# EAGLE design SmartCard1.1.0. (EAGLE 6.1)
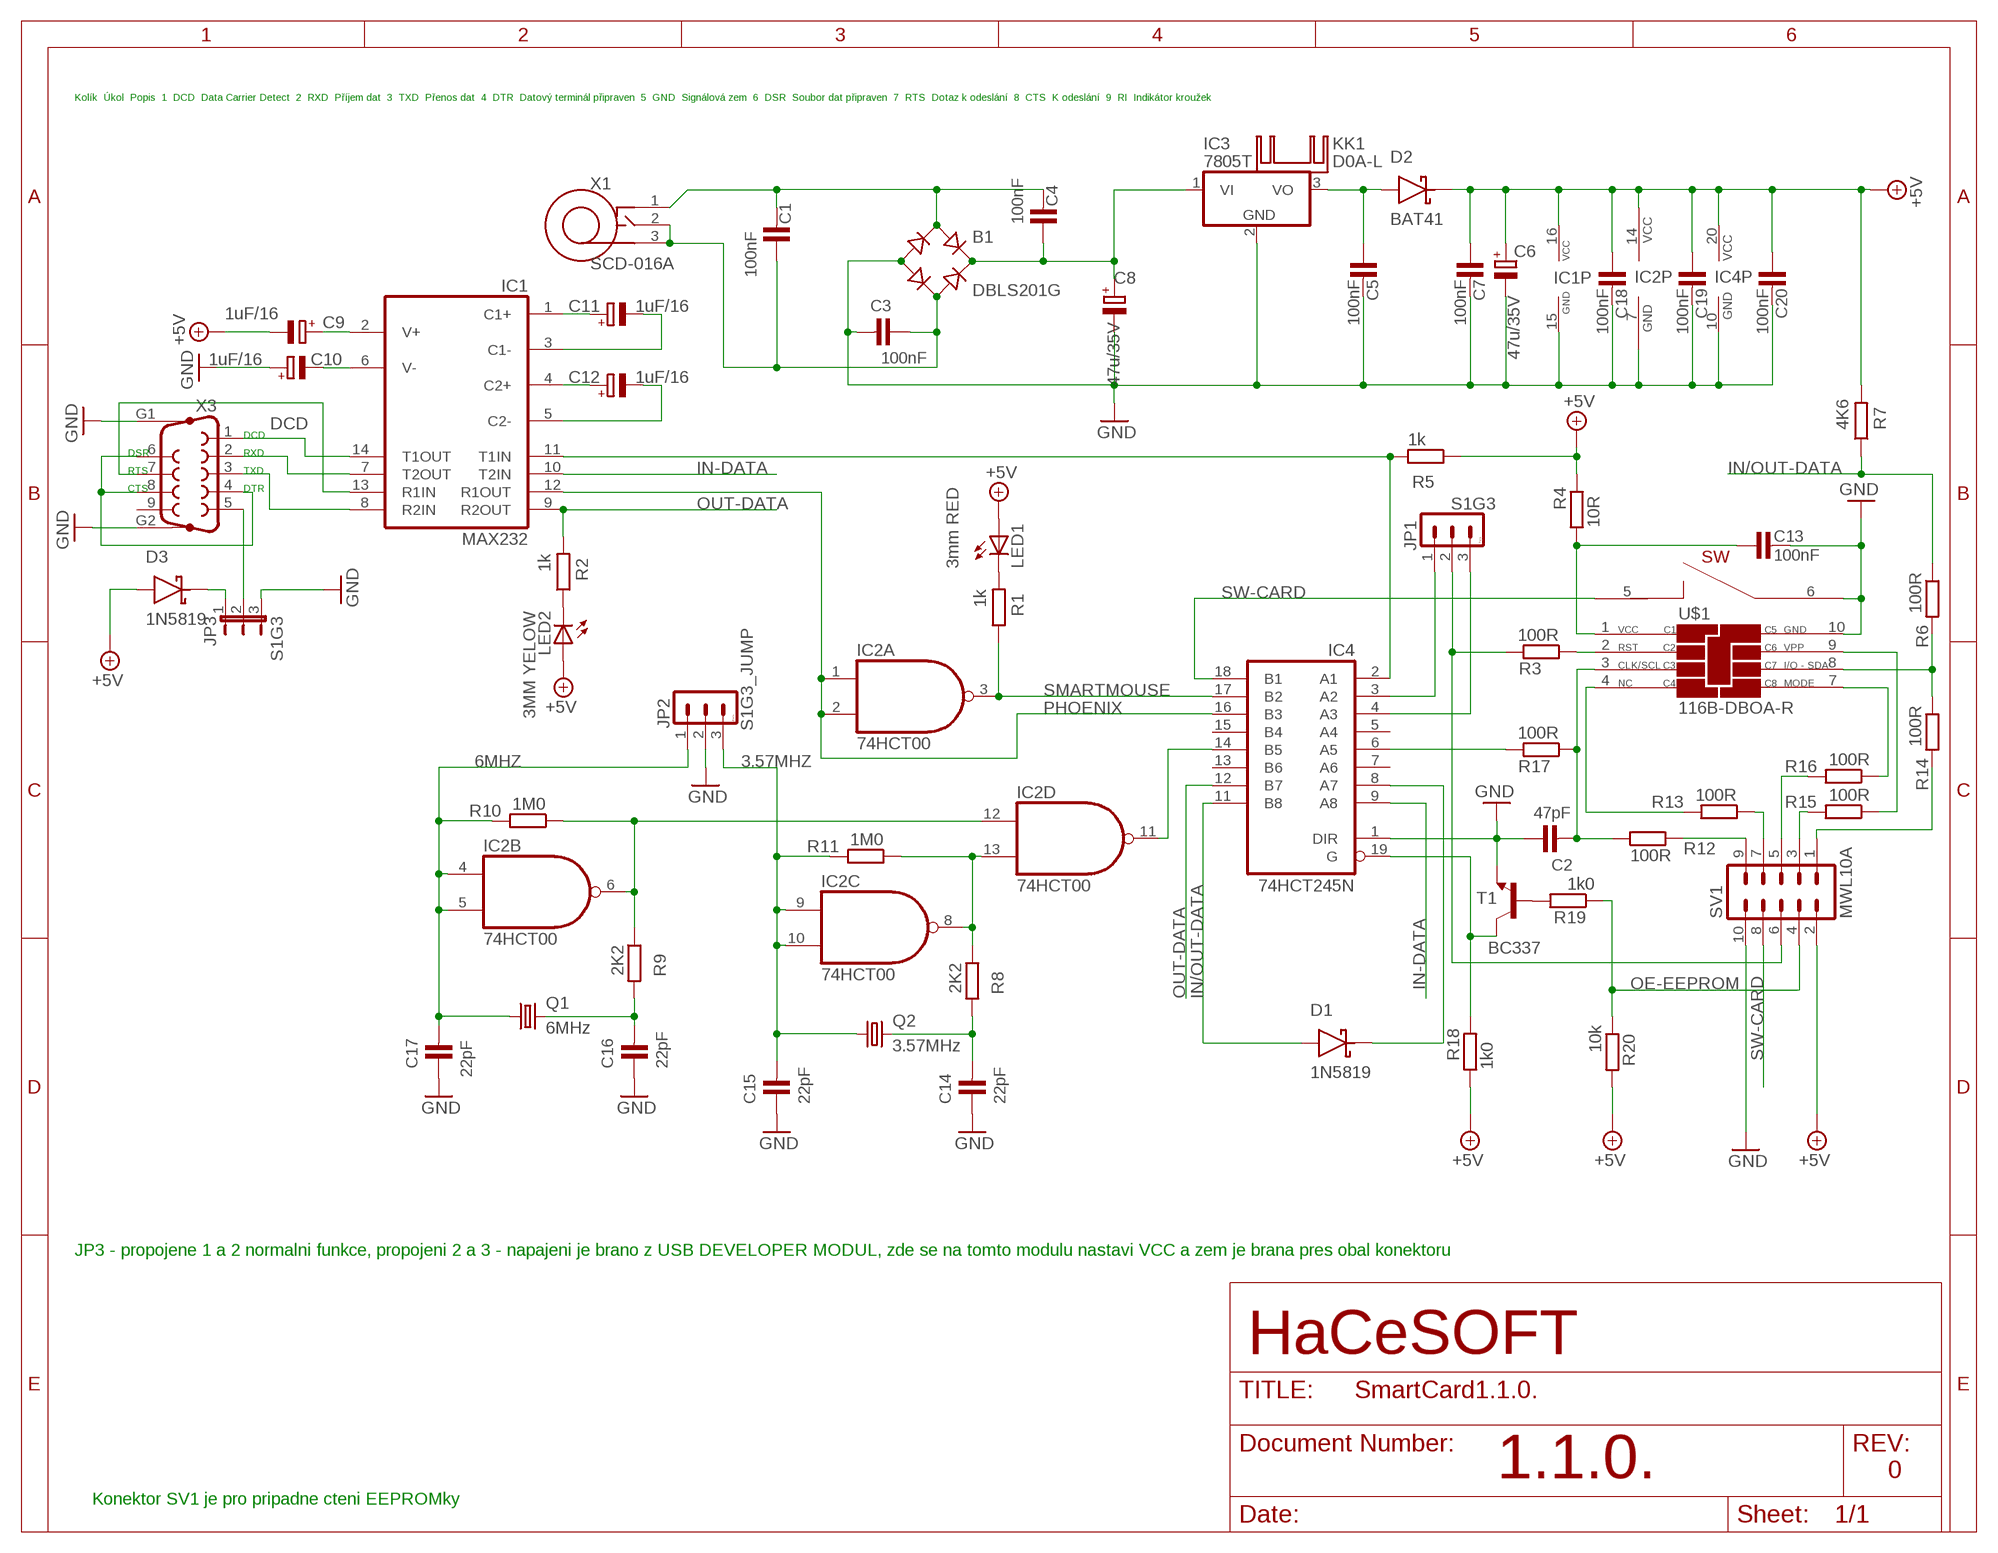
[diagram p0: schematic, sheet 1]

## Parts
B1  DBLS201G  [DBS]
C1  100nF  C-KERAMIK_SMD_1206  [1206]
C2  47pF  C-KERAMIK_SMD_1206  [1206]
C3  100nF  C-KERAMIK_SMD_1206  [1206]
C4  100nF  C-KERAMIK_SMD_1206  [1206]
C5  100nF  C-KERAMIK_SMD_1206  [1206]
C6  47u/35V  CPOL-EUE2.5-5  [E2,5-5]
C7  100nF  C-KERAMIK_SMD_1206  [1206]
C8  47u/35V  CPOL-EUE2.5-5  [E2,5-5]
C9  1uF/16  CPOL-EUSMCB  [SMC_B]
C10  1uF/16  CPOL-EUSMCB  [SMC_B]
C11  1uF/16  CPOL-EUSMCB  [SMC_B]
C12  1uF/16  CPOL-EUSMCB  [SMC_B]
C13  100nF  C-KERAMIK_SMD_1206  [1206]
C14  22pF  C-KERAMIK_SMD_1206  [1206]
C15  22pF  C-KERAMIK_SMD_1206  [1206]
C16  22pF  C-KERAMIK_SMD_1206  [1206]
C17  22pF  C-KERAMIK_SMD_1206  [1206]
C18  100nF  C-KERAMIK_SMD_1206  [1206]
C19  100nF  C-KERAMIK_SMD_1206  [1206]
C20  100nF  C-KERAMIK_5  [C-5]
D1  1N5819  BAT47  [DO35]
D2  BAT41  BAT47  [DO35]
D3  1N5819  BAT47  [DO35]
IC1  MAX232  [DIL16]
IC2  74HCT00  7400N  [DIL14]
IC3  7805T  [TO220H]
IC4  74HCT245N  [DIL20]
JP1  S1G3  S1G3_JUMP  [S1G3_JUM]
JP2  S1G3_JUMP  [S1G3_JUM]
JP3  S1G3  JP2E  [JP2]
KK1  D0A-L  [D02A-L]
LED1  3mm RED  LED3MM  [LED3MM]
LED2  3MM YELOW  LED3MM  [LED3MM]
Q1  6MHz  CSM-7X-DU  [CSM-7X-DU]
Q2  3.57MHz  CSM-7X-DU  [CSM-7X-DU]
R1  1k  R-EU_M1206  [M1206]
R2  1k  R-EU_0204/7  [0204/7]
R3  100R  R-EU_0204/7  [0204/7]
R4  10R  R-EU_0204/7  [0204/7]
R5  1k  R-EU_M1206  [M1206]
R6  100R  R-EU_M1206  [M1206]
R7  4K6  R-EU_0204/7  [0204/7]
R8  2K2  R-EU_M1206  [M1206]
R9  2K2  R-EU_M1206  [M1206]
R10  1M0  R-EU_M1206  [M1206]
R11  1M0  R-EU_M1206  [M1206]
R12  100R  R-EU_0204/7  [0204/7]
R13  100R  R-EU_0204/7  [0204/7]
R14  100R  R-EU_M1206  [M1206]
R15  100R  R-EU_M1206  [M1206]
R16  100R  R-EU_M1206  [M1206]
R17  100R  R-EU_0204/7  [0204/7]
R18  1k0  R-EU_M1206  [M1206]
R19  1k0  R-EU_0204/7  [0204/7]
R20  10k  R-EU_M1206  [M1206]
SV1  MWL10A  ML10L  [ML10L]
T1  BC337  [TO92]
U$1  116B-DBOA-R  [693030010810]
X1  SCD-016A  NAPAJECI_KONEKTOR_SCD-016A  [NAPAJECI_KONEKTOR_SCD-016A]
X3  F09HP  [F09HP]

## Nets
3.57MHZ: C15.2 IC2.9(C:I0) IC2.10(C:I1) JP2.3 Q2.1 R11.2
6MHZ: C17.2 IC2.4(B:I0) IC2.5(B:I1) JP2.1 Q1.1 R10.2
+5V: C6.+ C7.1 C9.- C18.1 C19.1 C20.1 D2.K D3.A IC1.16(VCC) IC2.14(P:VCC) IC4.20(VCC) LED1.A LED2.A R4.2 R5.1 R7.2 R18.1 R20.2 SV1.2
DCD: IC1.14(T1OUT) X3.1
DTR: X3.4 X3.6 X3.8
GND: B1.- C2.1 C3.2 C5.2 C6.- C7.2 C8.- C10.+ C13.2 C14.1 C15.1 C16.1 C17.1 C18.2 C19.2 C20.2 IC1.15(GND) IC2.7(P:GND) IC3.2(GND) IC4.1(DIR) IC4.10(GND) JP2.2 JP3.3 SV1.10 T1.1(E) U$1.6(SWITCH2) U$1.10(GND) X3.G1 X3.G2
IN-DATA: IC1.10(T2IN) IC4.9(A8)
IN/OUT-DATA: D1.A IC4.11(B8) R6.1 R7.1
IN/OUT-DATA-X: D1.K IC4.8(A7)
N$5: IC1.13(R1IN) X3.7
N$6: JP3.2 X3.5
N$7: B1.+ C4.1 C8.+ IC3.1(VI)
N$8: C9.+ IC1.2(V+)
N$9: B1.AC1 C1.2 C4.2 X1.1(OBAL)
N$10: D3.K JP3.1
N$11: C5.1 D2.A IC3.3(VO)
N$12: C10.- IC1.6(V-)
N$13: C11.+ IC1.1(C1+)
N$14: C12.+ IC1.4(C2+)
N$15: C11.- IC1.3(C1-)
N$16: C12.- IC1.5(C2-)
N$17: LED1.K(C) R1.2
N$19: IC4.19(G) R18.2 T1.3(C)
N$20: LED2.K(C) R2.1
N$21: JP1.2 R3.2 SV1.6
N$22: R3.1 U$1.2(RST)
N$23: IC4.3(A2) JP1.1
N$24: R6.2 R14.1 U$1.8(I/O-SDA)
N$25: IC1.11(T1IN) IC4.2(A1) R5.2
N$26: IC2.11(D:O) IC4.14(B5)
N$27: IC2.6(B:O) IC2.12(D:I0) R9.1 R10.1
N$28: C16.2 Q1.2 R9.2
N$29: C2.2 R12.1 R17.1 U$1.3(CLK/SCL)
N$30: IC2.8(C:O) IC2.13(D:I1) R8.1 R11.1
N$31: C14.2 Q2.2 R8.2
N$32: R12.2 SV1.9
N$33: R19.2 T1.2(B)
N$34: C13.1 R4.1 U$1.1(VCC)
N$35: R13.1 SV1.7
N$36: R13.2 U$1.4(NC)
N$37: R14.2 SV1.1
N$38: R15.1 U$1.9(VPP)
N$39: R16.1 U$1.7(MODE)
N$40: R15.2 SV1.3
N$41: R16.2 SV1.5
N$42: B1.AC2 C1.1 C3.1 X1.2 X1.3(PROSTREDEK)
N$43: IC4.4(A3) JP1.3
N$46: IC4.6(A5) R17.2
OE-EEPROM: R19.1 R20.1 SV1.4
OUT-DATA: IC1.9(R2OUT) IC4.12(B7) R2.2
PHOENIX: IC1.12(R1OUT) IC2.1(A:I0) IC2.2(A:I1) IC4.16(B3)
RXD: IC1.7(T2OUT) X3.2
SMARTMOUSE: IC2.3(A:O) IC4.17(B2) R1.1
SW-CARD: IC4.18(B1) SV1.8 U$1.5(SWITCH1)
TXD: IC1.8(R2IN) X3.3
Unconnected: IC4.5(A4) IC4.7(A6) IC4.13(B6) IC4.15(B4) X3.9

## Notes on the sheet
- Kolík  Úkol  Popis  1  DCD  Data Carrier Detect  2  RXD  Příjem dat  3  TXD  Přenos dat  4  DTR  Datový terminál připraven  5  GND  Signálová zem  6  DSR  Soubor dat připraven  7  RTS  Dotaz k odeslání  8  CTS  K odeslání  9  RI  Indikátor kroužek
- DCD
- DSR | RXD
- RTS | TXD
- CTS | DTR
- JP3 - propojene 1 a 2 normalni funkce, propojeni 2 a 3 - napajeni je brano z USB DEVELOPER MODUL, zde se na tomto modulu nastavi VCC a zem je brana pres obal konektoru
- HaCeSOFT
- 1.1.0. | 0
- Konektor SV1 je pro pripadne cteni EEPROMky

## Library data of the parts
B1 = rectifier:DB?*G: Single Phase 1.0 AMP Glass Passivated Bridge Rectifier Taiwan Semiconductor Co.,Ltd. - TSC Source: http://www.taiwansemi.com/TSCbig5/ezcatfiles/cust/img/img/db101g.pdf http://www.ts.com.tw/db/pictures/modules/PDT/PDT060207001/DBLS201G.pdf
C1-C5 C7 C13-C20 = #hacesoft:C-KERAMIK: Kondenzator - keramicky
C6 C8-C12 = rcl:CPOL-EU: POLARIZED CAPACITOR, European symbol
D1-D3 = #_GM99:BAT47
IC1 = maxim:MAX232: RS232 TRANSEIVER; MF: MAXIM; MPN: MAX232ACPE+; OC_FARNELL: 9723773; OC_NEWARK: 68K4544
IC2 = 74xx-us:74*00: Quad 2-input NAND gate
IC3 = linear:78*: Positive VOLTAGE REGULATOR Source: http://cache.national.com/ds/LM/LM78L05.pdf http://www.fairchildsemi.com/ds/LM/LM7805.pdf
IC4 = 74xx-eu:74*245: Octal BUS TRANSCEIVER, 3-state
JP1 JP2 = #PaJa_konektory:S1G3_JUMP: Radove konektory - koliky - 3x
JP3 = #hacesoft:JP2E: JUMPER
KK1 = heatsink:D0A-L: HEATSINK
LED1 LED2 = led:LED: LED
Q1 Q2 = crystal:CSM-7X-DU: SMD CRYSTAL; OC_FARNELL: unknown; OC_NEWARK: unknown
R1-R20 = resistor:R-EU_: RESISTOR, European symbol
SV1 = con-ml:ML10L: HARTING; OC_FARNELL: unknown; OC_NEWARK: unknown
T1 = transistor:BC337: NPN TRANSISTOR
U$1 = Smart Card Socket Through Hole Type, Single Port:116B-DBOA-R
X1 = #hacesoft:NAPAJECI_KONEKTOR_SCD-016A
X3 = con-subd:F09HP: SUB-D; OC_FARNELL: unknown; OC_NEWARK: unknown

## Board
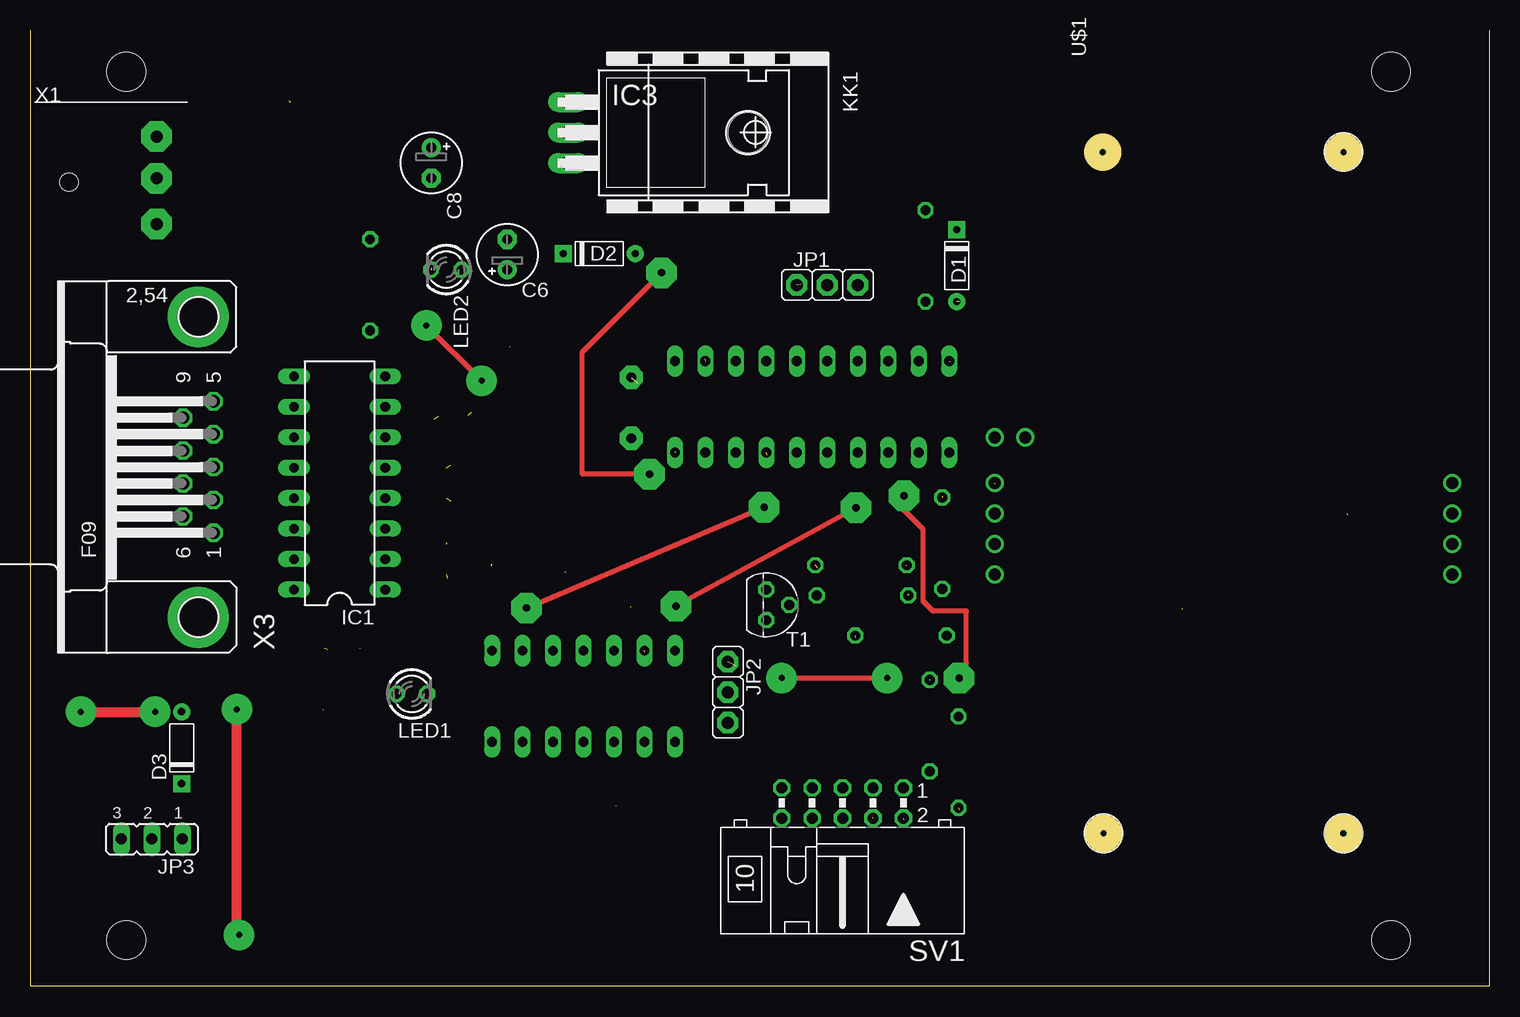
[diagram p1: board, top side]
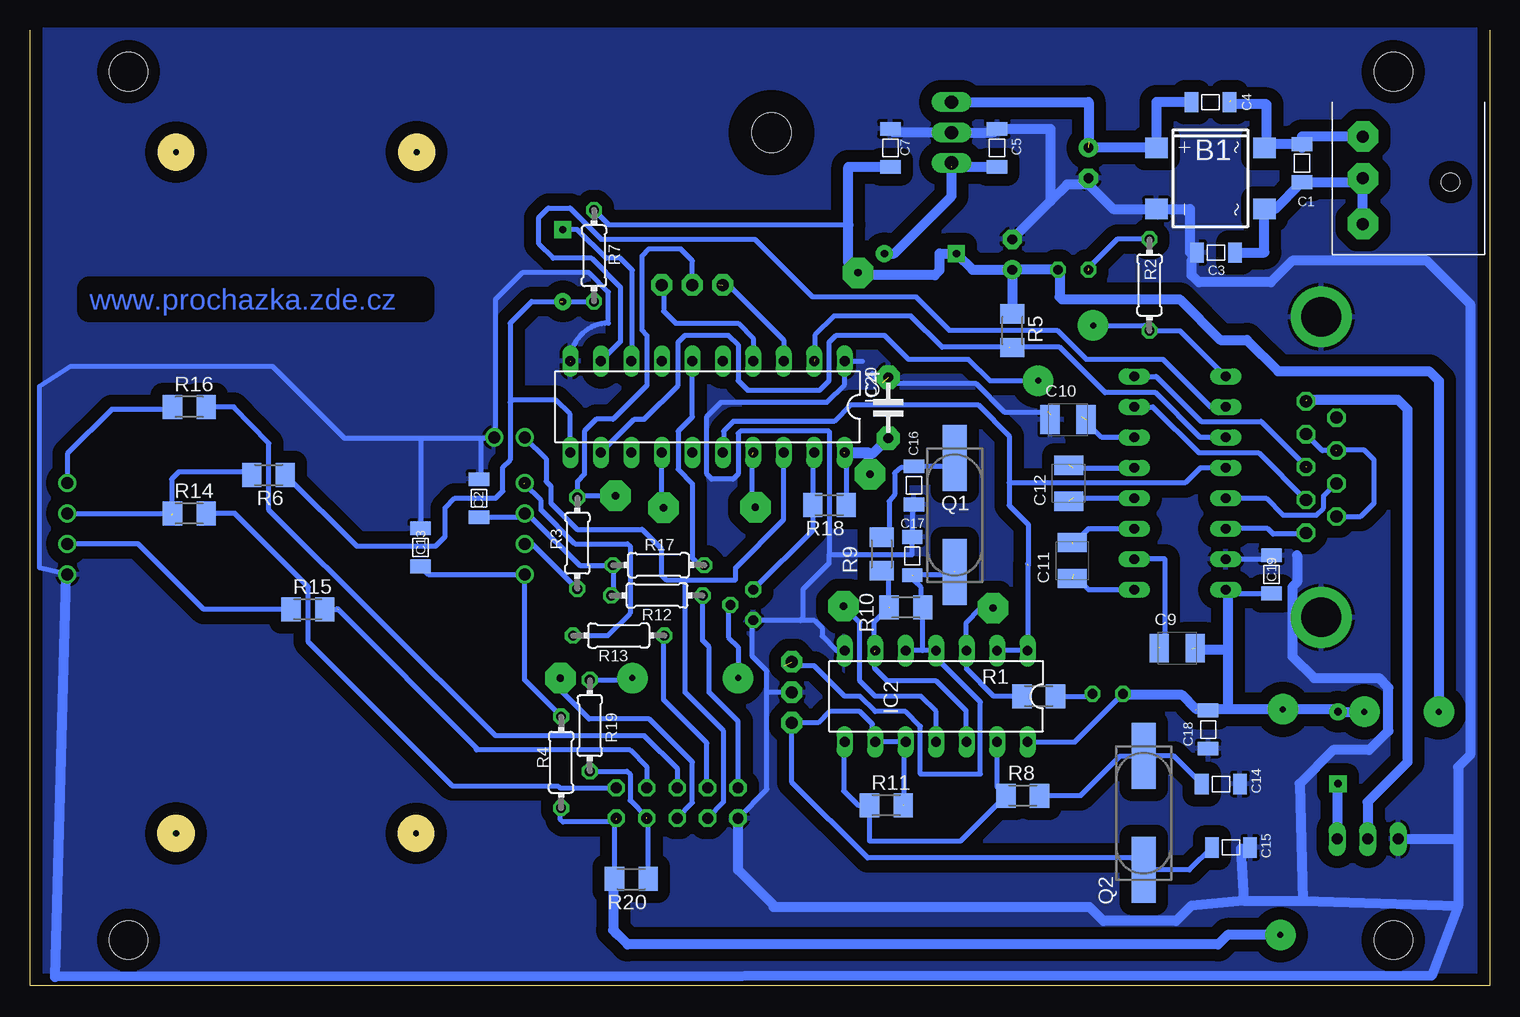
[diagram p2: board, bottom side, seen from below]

Size 121.63 x 79.68 mm. Coordinates in mm from the lower left corner, seen from the top.
Outline: 121.63,79.68 121.63,0 0,0 0,79.68
Copper layers (1*16): Top 0.035mm / dielectric 1.5mm / Bottom 0.035mm
Design rules: minimum track width 10mil, minimum drill 12mil, track to track 8mil, track to pad 8mil, pad to pad 8mil, via to via 8mil, smd to smd 8mil, copper to edge 40mil, drill to drill 8mil, minimum pad ring 10mil, minimum via ring 8mil, stop-mask expansion 4mil, vias tented up to drill 0mil, thermal gap 10mil
Holes 3.2 mm at 113.43,3.81 113.43,76.2 8.02,3.81 8.02,76.2

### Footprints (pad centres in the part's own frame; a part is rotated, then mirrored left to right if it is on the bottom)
DBS = smd 1.7 x 1.9: + -2.55,-4.5; - 2.55,-4.5; AC1 -2.55,4.5; AC2 2.55,4.5
1206 = smd 1.143 x 1.702: 1 -1.587,0; 2 1.587,0
E2,5-5 = drill 0.813 pad 1.6: + -1.27,0 | drill 0.813 pad 1.6 octagon: - 1.27,0
SMC_B = smd 1.6 x 2.4: + -1.5,0; - 1.5,0
C-5 = drill 0.813 pad 1.93 octagon: 1 -2.54,0; 2 2.54,0
DO35 = drill 0.61 pad 1.422: A 6,0 | drill 0.61 pad 1.422 square: K 0,0
DIL16 = drill 0.813 long: 1 -8.89,-3.81; 2 -6.35,-3.81; 3 -3.81,-3.81; 4 -1.27,-3.81; 5 1.27,-3.81; 6 3.81,-3.81; 7 6.35,-3.81; 8 8.89,-3.81; 9 8.89,3.81; 10 6.35,3.81; 11 3.81,3.81; 12 1.27,3.81; 13 -1.27,3.81; 14 -3.81,3.81; 15 -6.35,3.81; 16 -8.89,3.81
DIL14 = drill 0.813 long: 1 -7.62,-3.81; 2 -5.08,-3.81; 3 -2.54,-3.81; 4 0,-3.81; 5 2.54,-3.81; 6 5.08,-3.81; 7 7.62,-3.81; 8 7.62,3.81; 9 5.08,3.81; 10 2.54,3.81; 11 0,3.81; 12 -2.54,3.81; 13 -5.08,3.81; 14 -7.62,3.81
TO220H = drill 1.118 long: 1 -2.54,-10.16; 2 0,-10.16; 3 2.54,-10.16 | hole 3.302: 0,4.826
DIL20 = drill 0.813 long: 1 -11.43,-3.81; 2 -8.89,-3.81; 3 -6.35,-3.81; 4 -3.81,-3.81; 5 -1.27,-3.81; 6 1.27,-3.81; 7 3.81,-3.81; 8 6.35,-3.81; 9 8.89,-3.81; 10 11.43,-3.81; 11 11.43,3.81; 12 8.89,3.81; 13 6.35,3.81; 14 3.81,3.81; 15 1.27,3.81; 16 -1.27,3.81; 17 -3.81,3.81; 18 -6.35,3.81; 19 -8.89,3.81; 20 -11.43,3.81
S1G3_JUM = drill 1.016 pad 1.778 octagon: 1 -2.54,0; 2 0,0; 3 2.54,0
JP2 = drill 0.914 long: 1 -2.54,0; 2 0,0; 3 2.54,0
LED3MM = drill 0.813 octagon: A -1.27,0; K 1.27,0
CSM-7X-DU = smd 5.5 x 2: 1 -4.75,0; 2 4.75,0
M1206 = smd 1.6 x 2: 1 -1.4,0; 2 1.4,0
0204/7 = drill 0.813 octagon: 1 -3.81,0; 2 3.81,0
ML10L = drill 0.914 octagon: 1 -5.08,-1.27; 2 -5.08,1.27; 3 -2.54,-1.27; 4 -2.54,1.27; 5 0,-1.27; 6 0,1.27; 7 2.54,-1.27; 8 2.54,1.27; 9 5.08,-1.27; 10 5.08,1.27
TO92 = drill 0.813 octagon: 1 1.27,0; 2 0,1.905; 3 -1.27,0
693030010810 = drill 1: 1 0,38.1; 2 2.54,38.1; 3 5.08,38.1; 4 7.62,38.1; 5 11.43,38.1; 6 11.43,35.56; 7 7.62,0; 8 5.08,0; 9 2.54,0; 10 0,0 | drill 0.5 pad 3: P$1 -21.594,29.048; P$2 -21.589,9.053; P$3 35.213,9.05; P$4 35.213,29.097
NAPAJECI_KONEKTOR_SCD-016A = drill 1 pad 2.54 octagon: 1 0,7.303; 2 0,3.81; 3 0,0 | hole 1.5: -7.303,3.493
F09HP = drill 1.016 octagon: 1 -5.486,-1.27; 2 -2.743,-1.27; 3 0,-1.27; 4 2.743,-1.27; 5 5.486,-1.27; 6 -4.115,1.27; 7 -1.372,1.27; 8 1.372,1.27; 9 4.115,1.27 | drill 3.302 pad 5.08: G1 -12.522,0; G2 12.522,0

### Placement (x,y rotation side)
B1  23.26,67.31 270 bottom
C1  15.64,68.58 90 bottom
C2  84.22,40.64 270 bottom
C3  22.8,61.12 180 bottom
C4  23.26,73.66 0 bottom
C5  41.04,69.85 90 bottom
C6  39.77,60.96 90 top
C7  49.93,69.85 90 bottom
C8  33.43,68.59 270 top
C9  26.03,28.14 0 bottom
C10  35.13,47.19 0 bottom
C11  34.78,35.44 90 bottom
C12  35.08,41.89 90 bottom
C13  89.09,36.54 90 bottom
C14  22.39,16.81 180 bottom
C15  21.54,11.53 180 bottom
C16  47.97,41.71 90 bottom
C17  48.11,35.82 270 bottom
C18  23.45,21.36 270 bottom
C19  18.18,34.29 90 bottom
C20  50.11,48.18 90 bottom
D1  77.23,63.04 270 top
D2  44.43,61.04 0 top
D3  12.63,16.84 90 top
IC1  25.8,41.91 90 top
IC2  46.12,24.13 180 bottom
IC3  55.01,71.12 270 top
IC4  65.17,48.26 180 bottom
JP1  66.44,58.42 0 top
JP2  58.15,24.46 270 top
JP3  10.16,12.23 180 top
KK1  55.01,71.12 180 top
LED1  31.82,24.33 0 top
LED2  34.69,59.69 180 top
Q1  44.58,39.24 90 bottom
Q2  28.83,14.39 90 bottom
R1  37.57,24.13 0 bottom
R2  28.34,58.42 270 bottom
R3  76.02,36.89 90 bottom
R4  77.37,18.63 270 bottom
R5  39.77,54.61 270 bottom
R6  101.75,42.58 180 bottom
R7  74.63,60.85 90 bottom
R8  38.9,15.84 0 bottom
R9  50.66,35.99 90 bottom
R10  48.64,31.53 0 bottom
R11  50.27,15.04 0 bottom
R12  69.38,32.53 0 bottom
R13  72.58,29.19 180 bottom
R14  108.35,39.37 0 bottom
R15  98.48,31.38 0 bottom
R16  108.35,48.26 0 bottom
R17  69.25,35.06 0 bottom
R18  55.01,40.06 180 bottom
R19  74.98,21.68 90 bottom
R20  71.52,8.89 180 bottom
SV1  67.71,15.24 180 top
T1  61.36,31.75 270 top
U$1  118.51,34.29 90 top
X1  10.56,63.5 0 top
X3  14.03,43.24 90 top

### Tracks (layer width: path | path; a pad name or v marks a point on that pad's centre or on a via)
3.57MHZ  (1 unrouted)
  Bottom 0.406: 48.83,15.04 48.83,20.15 IC2.10 IC2.9 51.43,20.55 51.43,21.82 52.47,22.86 55.01,22.86 55.95,21.92 JP2.3 58.15,16.96 51.83,10.64 29.83,10.64 Q2.1 25.02,9.64 C15.2
6MHZ  (3 unrouted)
  Bottom 0.406: IC2.4 IC2.5 48.83,27.94 48.83,27.84 | JP2.1 57.99,26.84 | IC2.4 46.12,27.33 42.43,23.64 42.43,17.64 47.43,17.64 47.43,21.63 48.66,22.86 51.2,22.86 52.47,24.13 53.74,24.13 56.28,26.67 58.82,26.67 | IC2.4 47.24,27.94 R10.2 47.38,31.67 47.38,33.19 47.98,33.79 47.98,34.14 48.03,34.19 47.93,34.29 44.68,34.29 44.63,34.34 44.63,34.49
+5V  (via drill 0.5 pad 2.54, 0.6 pad 2.54)  (5 unrouted)
  Top 0.406: v51.63,42.64 46.03,42.64 46.03,52.84 v52.63,59.44
  Top 0.813: v4.23,22.84 v10.43,22.84 | v17.43,4.24 17.23,4.24 v17.23,23.04
  Bottom 0.406: IC1.16 21.99,32.7 C19.1 | R20.2 72.92,13.75 | 72.92,13.75 72.83,13.84 | 72.92,13.75 73.03,13.64 77.23,13.64 77.43,13.84 77.43,14.64 | C6.+ 39.83,59.63 | R5.1 40,56.24 | IC4.20 53.61,44.45 R18.1 | R7.2 73.41,63.44 53.43,63.44 | v51.63,42.64 51.43,42.84 | C18.1 24.48,22.95 24.48,23.14 | IC2.14 34.56,20.32 LED1.A 30.63,24.25 30.63,24.24
  Bottom 0.813: C7.1 53.41,68.26 53.43,68.24 53.43,63.44 53.43,60.24 v52.63,59.44 53.43,59.24 46.23,59.24 45.83,59.64 45.83,61.04 D2.K 43.08,59.69 C6.+ 36.06,59.69 36.01,59.64 | LED2.A 36.01,59.64 | 39.83,59.63 39.77,59.57 R5.1 | 36.01,59.64 35.83,59.46 35.83,57.44 35.63,57.24 25.83,57.24 22.43,53.84 20.23,53.84 17.63,51.24 5.03,51.24 4.23,50.44 v4.23,22.84 | v10.43,22.84 D3.A 12.83,23.04 v17.23,23.04 21.83,23.04 | 21.83,23.04 24.43,23.04 25.63,24.24 30.63,24.24 | 21.99,32.7 21.83,32.54 21.83,28.04 | 21.83,28.04 21.83,23.04 | 24.93,28.14 24.83,28.04 21.83,28.04 | R20.2 73.03,8.78 73.03,4.64 72.73,4.34 72.63,4.24 71.83,3.44 22.63,3.44 21.83,4.24 v17.43,4.24 | v51.63,42.64 51.73,42.64 51.73,44.44 53.83,44.44 53.83,44.39 51.36,44.39 C20.1
DCD
  Bottom 0.406: X3.1 15.41,37.64 18.03,37.64 18.49,38.1 IC1.14
DTR  (1 unrouted)
  Bottom 0.406: X3.6 10.75,39.12 9.63,40.24 9.63,43.84 10.43,44.64 12.83,44.64 | X3.8 13.93,44.61 X3.4
GND  (3 unrouted)
  Bottom 0.406: U$1.10 120.83,34.84 120.83,49.99 118.23,51.64 101.43,51.64 95.43,45.64 89.03,45.64 | 89.03,45.64 84.03,45.64 | 84.03,45.64 83.03,45.64 | 83.03,45.64 82.83,45.64 82.83,57.24 80.63,59.44 75.03,59.44 73.43,57.84 73.43,55.24 arc-90 76.63,52.04 | C13.2 89.03,38.19 89.03,45.64 | C2.1 84.03,42.42 84.03,45.64 | U$1.6 83.03,45.64 | 52.26,52.07 IC4.1 53.74,50.13 55.23,48.64 64.03,48.64 65.23,47.44 65.23,42.64 64.83,42.24 63.03,42.24 62.63,42.64 62.63,46.04 62.43,46.24 55.03,46.24 55.03,35.94 | 36.52,47.58 36.52,48.13 | 51.43,51.04 50.63,50.24 42.83,50.24 40.43,47.84 36.83,47.84 | SV1.10 60.23,16.37 60.23,24.44 | JP2.2 60.21,24.46 60.23,24.44 | 60.23,24.44 60.23,26.24 61.43,27.44 61.43,30.44 | 61.43,30.44 61.43,30.48 | 57.43,30.44 57.23,30.64 57.23,33.04 55.03,35.24 55.03,35.94 | 57.43,30.44 61.43,30.44 | 57.43,30.44 56.24,30.44 55.63,29.83 55.63,29.14 54.43,27.94 53.83,27.94 53.83,27.84 IC2.7 | IC1.15 18.18,35.56 C19.2 | 55.03,35.94 48.11,35.94 C17.1 48.11,40.12 C16.1 | C3.2 24.98,61.12 24.98,60.24 | 24.98,60.19 24.98,60.24 | 24.98,60.24 24.88,60.24 24.88,60.34
  Bottom 0.813: 20.72,11.43 20.47,7.09 | 20.47,7.09 15.58,7.09 | 15.58,7.09 2.63,6.64 | 24.83,60.44 24.83,59.24 24.23,58.64 18.23,58.64 16.43,60.44 5.23,60.44 1.63,56.84 1.63,19.24 2.63,18.24 2.63,12.04 | 59.63,6.64 62.63,9.64 62.63,13.84 | 2.63,6.64 4.83,0.84 119.53,0.74 118.63,34.24 | JP3.3 2.83,12.24 2.63,12.04 | 15.58,7.09 15.83,16.84 13.03,19.64 10.03,19.64 8.43,21.24 8.43,24.84 9.23,25.64 14.63,25.64 16.43,27.44 16.43,33.24 16.03,33.64 16.03,35.88 | 2.63,12.04 2.63,6.64 | 36.59,65.41 35.2,66.8 33.42,66.8 31.38,64.76 B1.- | 36.59,65.41 C6.- | C7.2 49.61,71.12 IC3.2 41.36,71.12 C5.2 36.59,71.44 36.59,65.41 | B1.- 27.43,64.76 27.43,64.69 | B1.- 24.98,64.76 24.98,61.12 | 20.47,7.09 24.88,6.64 26.13,5.39 32.18,5.39 33.33,6.54 59.68,6.54
  pour Bottom (isolate 1.016): 0.23,79.64 121.63,79.64 121.63,-0.16 0.23,-0.16
IN-DATA
  Bottom 0.406: IC4.9 72.43,53.7 72.43,58.24 74.83,60.64 78.03,60.64 79.23,61.84 79.23,64.04 78.43,64.84 76.63,64.84 74.03,62.24 61.23,62.24 56.43,57.44 47.83,57.44 45.03,54.64 36.03,54.64 33.63,52.24 27.23,52.24 23.25,48.26 IC1.10
IN/OUT-DATA  (1 unrouted)
  Bottom 0.406: R6.1 94.41,36.64 87.83,36.64 87.03,37.44 87.03,39.84 86.23,40.64 82.83,40.64 82.23,41.24 82.23,43.24 81.63,43.84 81.63,48.64 | 81.63,48.64 81.63,55.24 79.83,57.04 77.43,57.04 | IC4.11 76.63,44.48 76.63,47.64 77.83,48.84 81.43,48.84 81.63,48.64 | D1.A R7.1
IN/OUT-DATA-X
  Bottom 0.406: IC4.8 71.63,52.38 71.43,52.58 71.43,59.64 72.43,60.64 73.63,60.64 76.03,63.04 D1.K
N$5
  Bottom 0.406: IC1.13 18.63,40.64 17.23,39.24 14.43,39.24 13.83,39.84 13.83,40.84 12.8,41.87 X3.7
N$6  (1 unrouted)
  Bottom 0.813: JP3.2 10.16,15.31 6.83,18.64 6.83,48.04 7.63,48.84 15.23,48.84
N$7  (1 unrouted)
  Bottom 0.813: C4.1 27.76,73.66 B1.+ 32.92,69.86 33.42,70.36 33.42,73.66 IC3.1
N$8  (1 unrouted)
  Bottom 0.406: 27.47,28.14 27.03,28.58 27.03,35.56 IC1.2
N$9  (1 unrouted)
  Bottom 0.813: X1.1 15.64,70.8 C1.2 | C1.2 15.64,69.85 | C1.2 18.76,70.17 B1.AC1 18.58,69.86 18.58,73.49 21.58,73.49 21.58,73.79
N$10
  Bottom 0.813: D3.K 12.7,16.77 JP3.1
N$11  (1 unrouted)
  Bottom 0.813: C5.1 44.85,68.26 IC3.3 45.32,68.58 | D2.A 49.63,61.04 44.83,65.84 44.83,68.24 45.03,68.44 | 45.03,68.44 44.83,68.64 44.83,68.44 45.03,68.44
N$12  (1 unrouted)
  Bottom 0.406: IC1.6 32.31,45.72 34.03,47.44
N$13  (1 unrouted)
  Bottom 0.406: 34.69,34.29 33.42,33.02 IC1.1
N$14  (1 unrouted)
  Bottom 0.406: 34.69,40.64 IC1.4
N$15  (1 unrouted)
  Bottom 0.406: 34.69,36.83 33.42,38.1 IC1.3
N$16  (1 unrouted)
  Bottom 0.406: 34.69,43.18 IC1.5
N$17
  Bottom 0.406: R1.2 33.09,24.13 LED1.K
N$19
  Bottom 0.406: IC4.19 56.41,44.45 R18.2 56.41,37.97 T1.3
N$20  (2 unrouted)
  Bottom 0.406: 33.25,59.82 33.43,59.64 | R2.1 31.04,62.23 33.43,59.84
N$21  (via drill 0.6 pad 2.54)  (1 unrouted)
  Top 0.406: v77.43,25.64 78.03,26.84 78.03,31.24 75.23,31.24 74.43,32.04 74.43,38.04 72.83,39.64 v72.83,40.84
  Bottom 0.406: 66.63,58.61 JP1.2 66.43,60.44 67.43,61.44 70.03,61.44 70.63,60.84 70.63,54.64 70.23,54.24 70.23,50.04 73.03,47.24 74.43,47.24 75.43,46.24 75.43,42.64 76.02,42.05 R3.2 | SV1.6 66.43,15.25 66.43,18.64 70.03,22.24 75.03,22.24 77.23,24.44 v77.43,25.64 | v72.83,40.84 76.03,40.84
N$22
  Bottom 0.406: U$1.2 79.77,36.83 R3.1
N$23  (1 unrouted)
  Bottom 0.406: IC4.3 58.82,53.83 63.43,58.44 64.23,58.44
N$24  (1 unrouted)
  Bottom 0.406: U$1.8 R14.1 | R6.2 103.41,42.84 109.23,42.84 109.83,42.24 109.83,39.24
N$25  (2 unrouted)
  Bottom 0.406: IC1.11 24.11,45.72 27.83,49.44 32.03,49.44 35.83,53.24 40.03,53.24 | R5.2 39.77,53.04 39.97,53.24 45.63,53.24 48.23,55.84 54.63,55.84 56.23,54.24 56.23,52.24
N$26  (via drill 0.6 pad 2.54)
  Top 0.406: v53.83,31.64 v68.83,39.84
  Bottom 0.406: IC2.11 46.12,22.86 47.39,24.13 51.2,24.13 52.47,25.4 52.47,30.28 v53.83,31.64 | v68.83,39.84 68.98,39.99 IC4.14
N$27  (2 unrouted)
  Bottom 0.406: IC2.12 43.63,20.37 43.63,22.91 46.12,25.4 50.19,25.4 51.23,26.44 51.23,27.84 | IC2.6 51.28,27.94 51.28,30.34 50.13,31.49 50.13,31.54 50.08,31.59 50.08,34.44 50.51,34.44 R9.1
N$28
  Bottom 0.406: Q1.2 45.27,43.3 C16.2 47.58,43.19 49.03,43.19 49.58,42.74 49.58,40.94 50.03,40.39 50.03,37.44 50.13,37.34 50.61,37.34 R9.2
N$29  (2 unrouted)
  Bottom 0.406: U$1.3 80.41,39.05 | 80.41,39.05 C2.2 | 80.41,39.05 79.84,39.05 75.83,35.04 73.03,35.04 73.03,32.84 73.23,32.64
N$30
  Bottom 0.406: IC2.8 53.83,20.23 53.83,16.24 52.63,15.04 R11.1 51.67,12.08 51.63,12.04 44.1,12.04 R8.1 41.04,16.58 IC2.13
N$31
  Bottom 0.406: R8.2 34.09,15.84 30.79,19.14 Q2.2 26.31,19.14 C14.2
N$32
  Bottom 0.406: SV1.9 62.63,22.04 65.03,24.44 65.03,28.24 65.57,28.78 R12.2
N$33  (via drill 0.5 pad 2.54)  (1 unrouted)
  Top 0.406: v62.63,25.64 v71.43,25.64
  Bottom 0.406: T1.2 63.43,31.58 63.43,29.04 62.63,28.24 v62.63,25.64 | v71.43,25.64 71.63,25.44 75.03,25.44
N$34
  Bottom 0.406: C13.1 88.43,34.29 U$1.1 80.41,25.48 R4.1
N$35  (1 unrouted)
  Bottom 0.406: SV1.7 65.23,16.57 65.23,20.24 68.83,23.84 68.83,29.04
N$36  (1 unrouted)
  Bottom 0.406: 80.43,41.84 79.03,40.44 79.03,39.64 76.23,36.84 71.83,36.84 71.63,36.64 71.63,31.04 73.48,29.19 R13.2
N$37
  Bottom 0.406: 72.92,16.64 SV1.1 77.5,16.51 77.63,16.64 86.43,16.64 98.43,28.64 98.43,33.24 104.56,39.37 R14.2
N$38
  Bottom 0.406: R15.1 107.17,31.38 112.62,36.83 U$1.9
N$39
  Bottom 0.406: R16.1 109.97,48.04 114.83,48.04 118.51,44.36 U$1.7
N$40  (1 unrouted)
  Bottom 0.406: R15.2 95.97,31.38 | 96.03,31.44 84.43,19.84 84.43,19.64 71.63,19.64 70.25,18.26 SV1.3
N$41
  Bottom 0.406: R16.2 104.65,48.26 101.73,45.24 101.73,39.64 82.83,20.84 70.43,20.84 67.71,18.12 SV1.5
N$42
  Bottom 0.813: X1.3 X1.2 10.88,66.99 C1.1 17.87,64.76 B1.AC2 18.76,61.12 C3.1
N$43
  Bottom 0.406: JP1.3 68.83,58.27 68.83,56.24 67.83,55.24 62.63,55.24 61.36,53.97 IC4.4
N$46  (1 unrouted)
  Bottom 0.406: IC4.6 66.44,47.43 67.63,46.24 67.63,43.04 66.43,41.84 66.43,35.64 65.63,34.84 | 65.44,35.45 R17.2
OE-EEPROM  (1 unrouted)
  Bottom 0.406: R20.1 70.12,13.84 SV1.4 | R19.1 71.86,17.87 71.63,17.64 71.63,15.44 70.23,14.04 70.23,13.84
OUT-DATA  (via drill 0.5 pad 2.54)
  Top 0.406: v37.63,50.44 v33.03,55.04
  Bottom 0.406: 22.12,50.8 IC1.9 25.8,54.61 R2.2 28.77,55.04 v33.03,55.04 | IC4.12 71.27,47.24 70.43,47.24 67.63,50.04 67.63,53.64 67.03,54.24 63.43,54.24 62.63,53.44 62.63,50.44 61.83,49.64 55.83,49.64 55.03,50.44 55.03,53.64 54.43,54.24 50.43,54.24 48.43,52.24 43.43,52.24 41.63,50.44 v37.63,50.44
PHOENIX  (1 unrouted)
  Bottom 0.406: IC2.2 IC2.1 38.5,35.17 | IC1.12 24.09,43.18 25.36,41.91 40.03,41.91 | 40.03,41.91 40.03,45.84 42.63,48.44 53.23,48.44 54.63,47.04 63.03,47.04 63.83,46.24 63.83,44.52 IC4.16 | 40.03,41.91 40.03,40.04 38.43,38.44 38.43,35.04
RXD
  Bottom 0.406: IC1.7 28.05,48.26 24.23,44.44 19.24,44.44 X3.2
SMARTMOUSE  (via drill 0.6 pad 2.54)  (1 unrouted)
  Top 0.406: v41.38,31.49 v61.18,39.89
  Bottom 0.406: R1.1 41.32,24.13 43.58,26.39 IC2.3 43.63,27.99 43.63,30.24 42.43,31.44 v41.38,31.49 | v61.18,39.89 61.43,40.04 61.43,44.24
SW-CARD
  Bottom 0.406: SV1.8 63.83,15.31 63.83,21.24 67.03,24.44 67.03,33.84 | IC4.18 58.82,38.85 62.83,34.84 62.83,33.84 67.03,33.84 | U$1.5 78.63,43.94 78.63,42.04 78.23,41.64 78.23,40.24 76.03,38.04 70.63,38.04 69.03,36.44 69.03,34.24 68.63,33.84 67.03,33.84
TXD  (1 unrouted)
  Bottom 0.406: IC1.8 27.79,50.8 24.03,47.04 19.03,47.04 15.23,43.24

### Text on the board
Bottom: www.prochazka.zde.cz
